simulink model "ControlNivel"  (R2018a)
settings: Solver=VariableStepAuto  StartTime=0.0  StopTime=150  RelTol=1e-3
undefined symbols (not defined in the file): a6fa, ControlNivel, sdiscope

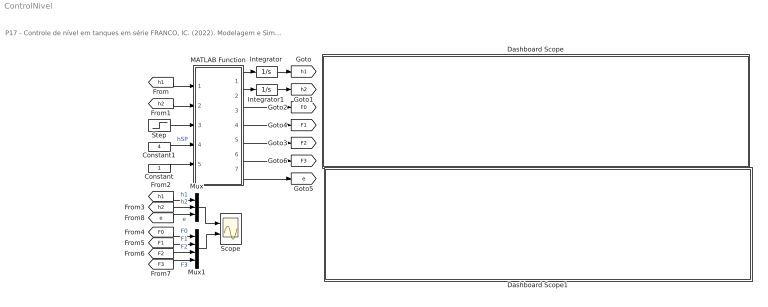
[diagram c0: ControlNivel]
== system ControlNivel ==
  note: P17 - Controle de nível em tanques em série FRANCO, IC. (2022). Modelagem e Simulação: Problemas Típicos da Engenharia Química para Simulação e Análise. NOTAS DE AULA INOVADORAS. The Journal of Engineering and Exact Sciences. Material Complementar.
  Constant : Constant
  Constant1 : Constant  Value=4
  Dashboard Scope : Subsystem  DialogController=hmiCreateDDGDialog  IsWebBlock=on  mask(MWDashboardBlock){webBlockId=23b581cc-3cc9-4af9-9a75-2e061a918594, webBlockType=sdiscope, ShowInitialText=on, HMISrcModelName=ControlNivel}
      mask prompts: webBlockId "WebBlock Id"; webBlockType "WebBlock Type"; HMISrcModelName "Source Model"
      mask help: SimulinkHMI:dialogs:HMIScopeDialogDesc
  Dashboard Scope1 : Subsystem  DialogController=hmiCreateDDGDialog  IsWebBlock=on  mask(MWDashboardBlock){webBlockId=33110f1a-1178-45ec-a6fa-1d1ec7dfb9c3, webBlockType=sdiscope, ShowInitialText=on, HMISrcModelName=ControlNivel}
      mask prompts: webBlockId "WebBlock Id"; webBlockType "WebBlock Type"; HMISrcModelName "Source Model"
      mask help: SimulinkHMI:dialogs:HMIScopeDialogDesc
  Integrator : Integrator  LimitOutput=on  UpperSaturationLimit=10  LowerSaturationLimit=0
  Integrator1 : Integrator  LimitOutput=on  UpperSaturationLimit=6  LowerSaturationLimit=0
  MATLAB Function : MATLAB Function  TreatAsAtomicUnit=on
  Mux : Mux  Inputs=3
  Mux1 : Mux
  Scope : Scope  NumInputPorts=2
  Step : Step  Time=70  Before=1  SampleTime=0
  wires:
  [h1] -> MATLAB Function/1(h1)
  MATLAB Function/4(F1) -> [F1]
  [h2] -> MATLAB Function/2(h2)
  Integrator/1 -> [h1]
  MATLAB Function/2(dh2) -> Integrator1/1
  MATLAB Function/1(dh1) -> Integrator/1
  Integrator1/1 -> [h2]
  Constant/1 -> MATLAB Function/5(KC)
  MATLAB Function/3(F0) -> [F0]
  MATLAB Function/5(F2) -> [F2]
  MATLAB Function/7(e) -> [e]
  [h1] -> Mux/1  "h1"
  [h2] -> Mux/2  "h2"
  MATLAB Function/6(F3) -> [F3]
  [F3] -> Mux1/4  "F3"
  [F2] -> Mux1/3  "F2"
  [F1] -> Mux1/2  "F1"
  [F0] -> Mux1/1  "F0"
  Constant1/1 -> MATLAB Function/4(hsp)  "hSP"
  Step/1 -> MATLAB Function/3("F3 ")
  [e] -> Mux/3  "e"
  Mux/1 -> Scope/1
  Mux1/1 -> Scope/2

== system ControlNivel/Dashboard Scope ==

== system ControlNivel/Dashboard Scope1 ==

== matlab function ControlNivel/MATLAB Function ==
function [dh1,dh2,F0,F1,F2,F3,e] = fcn(h1,h2,F3,hsp,KC)
%parâmetros
A1   =  4.00;
A2   =  3.00;
F0s  =  3.00;
K1   =  1.35;
K2   =  2.10;

%% equações auxiliares
F1=K1*sqrt(h1);
F2=K2*sqrt(h2);
%% controlador P
%error
e=hsp-h2;
%variável manipulada
F0=F0s+KC*e;

%% saturação
if F0<0
   F0=0;
end

%% modelo matemático
dh1=(F0-F1)/A1;
dh2=(F1+F3-F2)/A2;
end
